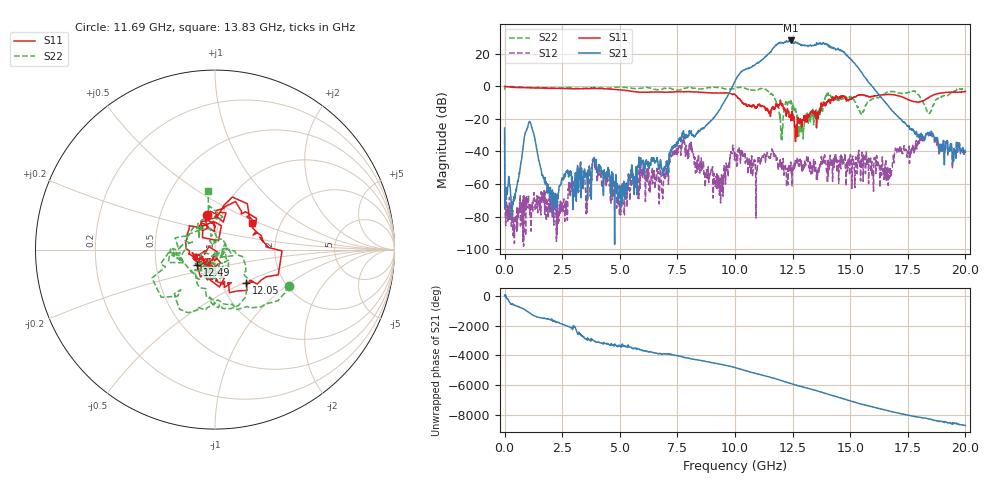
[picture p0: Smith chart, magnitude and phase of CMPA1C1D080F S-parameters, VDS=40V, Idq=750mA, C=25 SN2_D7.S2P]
!Keysight Technologies,E5071C,MY46632380,B.14.03
!Date: Tue Nov 10 06:00:56 2020
!Data & Calibration Information:
!Freq	S11:SOLT2(ON)	S21:SOLT2(ON)	S12:SOLT2(ON)	S22:SOLT2(ON)
!PortZ  Port1:50+j0  Port2:50+j0
!Above PortZ is port z conversion or system Z0 setting when saving the data.
!When reading, reference impedance value at option line is always used.
# Hz S dB R 50
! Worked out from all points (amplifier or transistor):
!   1601 points, 300 kHz to 20 GHz, reference 50 ohm
!   highest |S21| = 28.3 dB at 12.44 GHz (marker M1)
!   |S21| within 3 dB of that: 11.77 GHz to 12.88 GHz (1.118 GHz wide, 9.07 % of centre)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
!   unconditionally stable (mu >= 1): 12.74 MHz to 10.19 GHz; 10.2 GHz to end of sweep
!   at 3.325 GHz: K = 7498.08, MAG = -42.4 dB, |S12| = -52.4 dB
!   at 10 GHz: K = 5.08, MAG = 11.9 dB, |S12| = -40.7 dB
!   at 20 GHz: K = 1038.82, MAG = -33.3 dB, |S12| = -40.2 dB
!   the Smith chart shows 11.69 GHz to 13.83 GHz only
!   S11 on the Smith chart (normalised r, x): 11.69 GHz: 0.85, +0.34; 12.05 GHz: 1.31, -0.51; 12.49 GHz: 0.81, -0.14; 13.83 GHz: 1.43, +0.45
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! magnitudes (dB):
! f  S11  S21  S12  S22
! 300 kHz  0.0  -25.6  -32.7  -2.0
! 112.8 MHz  -0.2  -66.4  -79.5  -0.2
! 425.3 MHz  -0.6  -68.2  -96.6  -0.2
! 1.075 GHz  -0.8  -21.7  -76.7  -0.6
! 2.125 GHz  -1.2  -70.7  -81.6  -1.1
! 3.338 GHz  -1.4  -51.5  -50.4  -1.3
! 3.913 GHz  -1.3  -46.4  -49.0  -0.7
! 4.963 GHz  -2.0  -66.3  -72.4  -0.3
! 6.675 GHz  -3.4  -51.0  -55.5  -2.1
! 7.713 GHz  -3.2  -28.5  -32.9  -1.7
! 9.4 GHz  -4.0  -12.4  -59.3  -0.9
! 10 GHz  -5.1  3.2  -40.7  -1.0
! 11.69 GHz  -14.2  23.9  -43.8  -6.8
! 12.05 GHz  -11.9  26.9  -49.0  -25.9
! 12.44 GHz  -18.8  28.3  -49.2  -8.3
! 12.49 GHz  -17.7  26.6  -51.2  -14.3
! 12.86 GHz  -22.7  25.4  -47.0  -28.0
! 13.34 GHz  -15.1  24.9  -51.3  -15.6
! 13.83 GHz  -12.0  27.0  -46.2  -9.6
! 16.68 GHz  -4.9  -12.3  -51.9  -3.2
! 18.36 GHz  -7.2  -28.4  -28.8  -15.7
! 20 GHz  -3.1  -40.5  -40.2  -2.1
